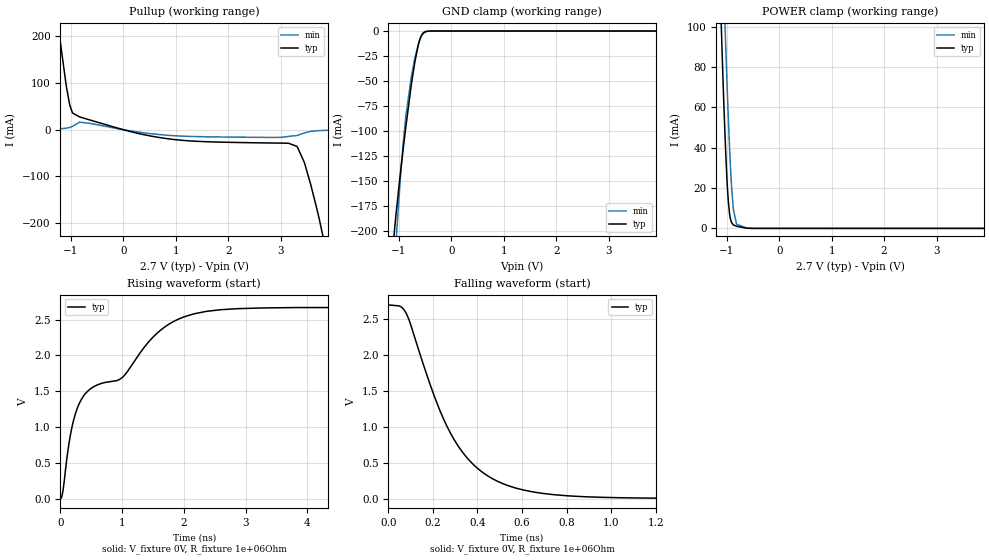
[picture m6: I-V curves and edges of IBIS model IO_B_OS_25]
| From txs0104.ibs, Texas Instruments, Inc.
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[Model]   IO_B_OS_25
Model_type   I/O_open_source
Polarity   Non-Inverting
Vinl=0.7
Vinh=1.7
Vmeas = 1.25
Vref = 0
Cref = 15pF
Rref = 1000000
|   typ   min   max
C_comp   11.90pF   11.90pF   11.90pF
[Voltage Range]   2.7   2.5   NA
[Temperature Range]   -40   27   NA
[Pullup Reference]   2.7   2.5   NA
[Pulldown Reference]   0   0   NA
[Power Clamp Reference]   2.7   2.5   NA
[GND Clamp Reference]   0   0   NA
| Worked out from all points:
|   slope of the pullup table from 0 to 0.405 V, typ, clamps not added: 36.9 ohm
|   GND clamp passes 1 mA (typ) near -0.51 V on its own axis
|   POWER clamp passes 1 mA (typ) near -0.80 V on its own axis
|   falling waveform, V_fixture 0V, R_fixture 1e+06Ohm: 20-80 % time 235ps typ, NA min, NA max; typ from 2.7 V to 0 V
|   rising waveform, V_fixture 0V, R_fixture 1e+06Ohm: 20-80 % time 1.3ns typ, NA min, NA max; typ from 0 V to 2.7 V
[GND Clamp]
|   Voltage   I(typ)   I(min)   I(max)
-2.5V     -1.514A    -1.588A    NA
-1.083V   -199mA     -234.7mA   NA
-1.052V   -182.6mA   -209.9mA   NA
-977.5mV  -145.6mA   -151.9mA   NA
-917.5mV  -118.1mA   -112.4mA   NA
-872.5mV  -98.31mA   -88.2mA    NA
-767.5mV  -55.83mA   -47.63mA   NA
-692.5mV  -30.2mA    -26.59mA   NA
-625mV    -12.91mA   -12.53mA   NA
-572.5mV  -4.84mA    -5.509mA   NA
-505mV    -845uA     -1.336mA   NA
4.992V    0A         0A         NA
[Pullup]
|   Voltage   I(typ)   I(min)   I(max)
-2.5V     1.44A      358.6uA    NA
-1.248V   228.3mA    1.762mA    NA
-1.09V    95.28mA    3.234mA    NA
-1.022V   52.82mA    4.786mA    NA
-970mV    35.87mA    7.072mA    NA
-835mV    27.44mA    16.18mA    NA
845mV     -19.35mA   -11.91mA   NA
3.312V    -35.89mA   -12.35mA   NA
3.462V    -74.65mA   -6.619mA   NA
3.732V    -190.5mA   -1.959mA   NA
3.822V    -237.6mA   -1.533mA   NA
4.992V    -1.311A    -379.1uA   NA
[POWER Clamp]
|   Voltage   I(typ)   I(min)   I(max)
-2.5V     1.44A      1.495A     NA
-1.127V   119.1mA    179mA      NA
-1.075V   76.33mA    134.3mA    NA
-1.03V    43.91mA    98.01mA    NA
-1V       26.19mA    75.33mA    NA
-970mV    13.34mA    54.45mA    NA
-940mV    6.065mA    36.14mA    NA
-910mV    2.974mA    21.39mA    NA
-872.5mV  1.71mA     9.23mA     NA
-812.5mV  1.054mA    2.051mA    NA
-587.5mV  66.64uA    102.2uA    NA
4.992V    0A         0A         NA
[Ramp]
R_load = 1e+06
|   typ   min   max
dV/dt_r   1.61995/1.30141e-09  NA   NA
dV/dt_f   1.61995/2.34702e-10  NA   NA
[Falling Waveform]
V_fixture = 0V
R_fixture = 1e+06Ohm
C_fixture = 0F
|   Time   V(typ)   V(min)   V(max)
0s        2.7V       NA         NA
53.73ps   2.678V     NA         NA
80.47ps   2.58V      NA         NA
243.6ps   1.141V     NA         NA
310.4ps   748.3mV    NA         NA
379.4ps   483mV      NA         NA
465.3ps   282.6mV    NA         NA
567.6ps   152.3mV    NA         NA
880.3ps   27.59mV    NA         NA
19.9ns    0V         NA         NA
[Rising Waveform]
V_fixture = 0V
R_fixture = 1e+06Ohm
C_fixture = 0F
|   Time   V(typ)   V(min)   V(max)
0s        0V         NA         NA
39.17ps   103.4mV    NA         NA
123.2ps   684.7mV    NA         NA
197.6ps   1.04V      NA         NA
390.1ps   1.451V     NA         NA
995.4ps   1.686V     NA         NA
1.419ns   2.178V     NA         NA
1.712ns   2.409V     NA         NA
2.358ns   2.613V     NA         NA
19.9ns    2.7V       NA         NA
